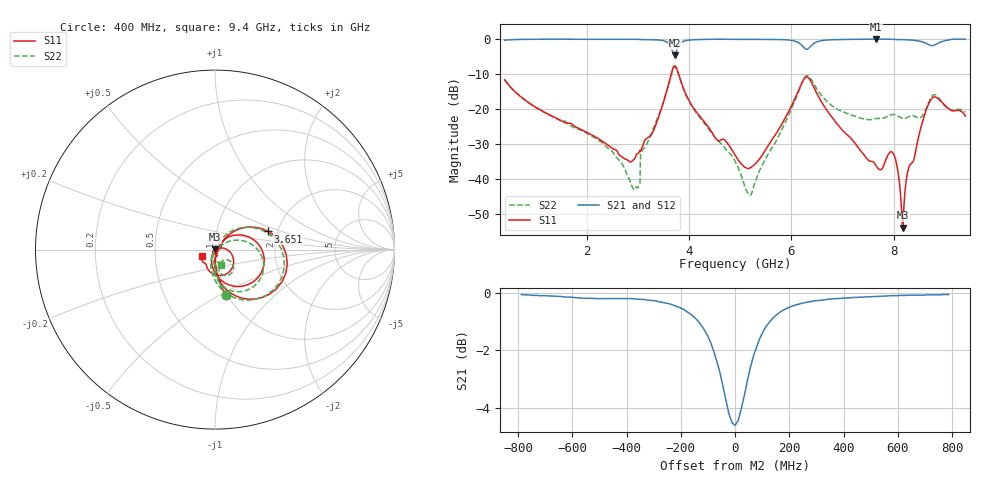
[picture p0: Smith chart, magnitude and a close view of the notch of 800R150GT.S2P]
!  American Technical Ceramics  Date:  6/19/09
!  One Norden Lane
!  Huntington Station,  NY.  11746-2102
!  Tel:  (631) 622-4700  Fax:  (631) 622-4748
!  Part Number  800R150GT
!  Description: Ultra-low ESR, NPO  Mounting Orientation: Horizontal
!  Application: High RF power Filters, Combiners, Matching networks,
!  Antenna, DC block, Bypass and Couplers
# GHZ S DB R 50
! Freq  |S11|  S11 Ph  |S21|  S21 Ph  |S12|  S12 Ph  |S22|  S22 Ph
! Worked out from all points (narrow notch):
!   801 points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, 400 MHz to 9.4 GHz, reference 50 ohm
!   highest |S21| = -0.01 dB at 7.645 GHz (marker M1); lowest = -4.6 dB at 3.719 GHz (marker M2)
!   notch at M2: 4.5 dB deep, 131 MHz wide at half that depth
!   lowest |S11| = -53.8 dB at 8.174 GHz (marker M3), VSWR 1.00, Z = 49.9 + j0.174 ohm
!   |S11| at or under -10 dB: start of sweep to 3.653 GHz; 3.799 GHz to end of sweep
!   |S22| runs from -44.5 to -7.9 dB; largest |S21 - S12| = 0.0027
!   S11 on the Smith chart (normalised r, x): 400 MHz: 0.98, -0.54; 3.651 GHz: 1.79, +0.40; 9.4 GHz: 0.86, -0.06
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0.4  -11.61 -76.4  -0.32 13.3  -0.33 13.3  -11.61 -76.7
1.908  -25.88 -87.5  -0.04 -6.0  -0.04 -6.0  -26.10 -102.7
2.493  -31.08 -72.8  -0.06 -10.0  -0.07 -10.0  -31.90 -117.3
2.954  -33.75 -2.4  -0.07 -13.6  -0.08 -13.5  -42.60 154.3
3.1  -30.16 27.8  -0.15 -14.9  -0.16 -14.9  -31.46 54.9
3.404  -22.39 47.8  -0.26 -18.9  -0.27 -18.9  -21.90 56.3
3.651  -10.08 18.8  -2.37 -28.8  -2.38 -28.9  -10.35 18.1
3.719  -7.62 -18.3  -4.62 -13.5  -4.63 -13.4  -7.90 -20.6
3.944  -15.83 -83.3  -0.42 -7.5  -0.42 -7.5  -16.00 -92.1
4.9  -33.03 -67.5  -0.08 -19.1  -0.08 -19.1  -34.76 -108.6
5.204  -36.65 -9.9  -0.09 -21.2  -0.09 -21.2  -44.50 -36.1
6.239  -11.61 -0.9  -2.32 -32.6  -2.33 -32.5  -11.50 -9.4
6.408  -12.78 -62.6  -1.60 -16.1  -1.60 -16.0  -11.95 -66.6
6.891  -24.13 -108.5  -0.15 -24.1  -0.15 -24.0  -19.98 -92.5
7.645  -35.82 -107.0  -0.01 -30.1  0.00 -30.0  -22.65 -75.0
7.904  -32.69 -87.7  -0.03 -32.4  -0.03 -32.3  -21.84 -68.7
8.039  -34.42 -133.1  -0.12 -33.5  -0.11 -33.4  -21.62 -72.9
8.174  -53.76 121.9  -0.18 -34.5  -0.17 -34.4  -22.55 -69.4
8.286  -37.01 7.5  -0.23 -35.5  -0.23 -35.4  -22.20 -61.8
8.534  -25.02 5.8  -0.71 -38.4  -0.70 -38.4  -22.27 -48.8
8.725  -17.28 -43.7  -1.84 -35.1  -1.83 -35.0  -16.73 -44.7
9.4  -21.96 -154.7  -0.01 -34.3  -0.01 -34.2  -20.80 -68.7
